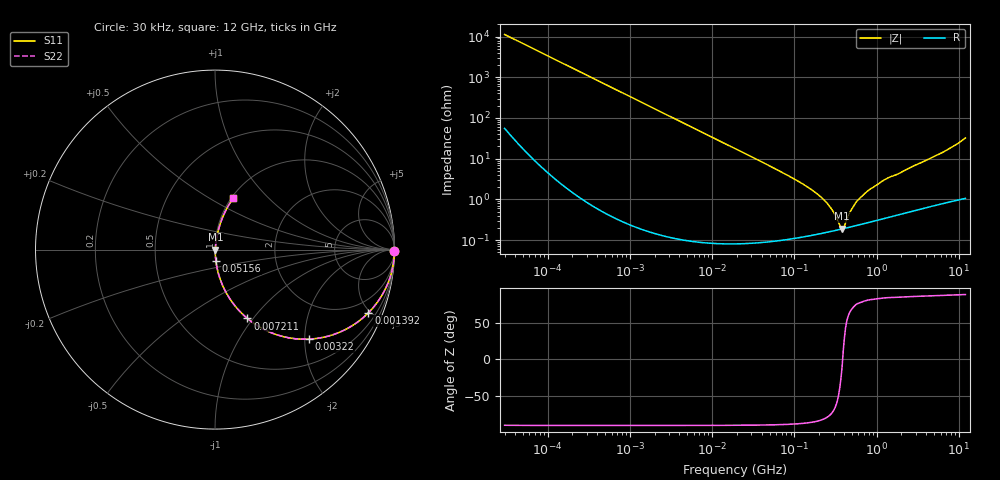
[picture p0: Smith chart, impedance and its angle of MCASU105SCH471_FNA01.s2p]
! MCASU105SCH471_FNA01  S-PARAMETER MODEL  ( General Type )
! Model Generated by TAIYO YUDEN Corporation (http://www.ty-top.com)
! Version 1.0
! TAIYO YUDEN Control No. 130207
! Copyright(c) 2013 TAIYO YUDEN CO.,LTD. All Rights Reserved.
! Product Description (link to TY-COMPAS)
! https://ds.yuden.co.jp/TYCOMPAS/or/detail?pn=MCASU105SCH471JFNA01&u=M
! Products Name : Multilayer Ceramic Capacitors
! Characteristics :
!  Capacitance : 470 pF , Rated Voltage : 50V , TCC : CH / C0H
!  Case Size : 1.0 x 0.5 / 0.039 x 0.02 [mm/inch] , Thickness : 0.5 / 0.02 [mm/inch]
!  (Conditions: Temperature = 25 degC , DC Bias Current/Voltage = 0A / 0V)
! External Node Assignments :
!  1  o---| |---o  2
! GND o---------o GND
! Frequency Range : 30000Hz  -  12GHz  [ 401 STEP ]
# MHz S RI R 50
! Freq[MHz].  S11 Real  S11 Imag  S21 Real  S21 Imag  S12 Real  S12 Imag  S22 Real  S22 Imag
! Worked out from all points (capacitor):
!   401 points, 30 kHz to 12 GHz, reference 50 ohm
!   read as one part in series: C = 471 pF near 32 kHz
!   lowest |Z| = 191 mohm at 380.7 MHz (marker M1)
!   series resonance near 386.2 MHz, so ESL is about 360 pH
!   S11 on the Smith chart (normalised r, x): 30 kHz: open; 1.392 MHz: 1.00, -4.86; 3.22 MHz: 1.00, -2.10; 7.211 MHz: 1.00, -0.94; 51.56 MHz: 1.00, -0.13; 12 GHz: 1.02, +0.65
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0.03  0.9999 -0.00887  0.000122 0.00887  0.000122 0.00887  0.9999 -0.00887
0.260295  0.994 -0.0765  0.00595 0.0765  0.00595 0.0765  0.994 -0.0765
0.730518  0.9553 -0.2064  0.0447 0.2064  0.0447 0.2064  0.9553 -0.2064
1.392304  0.8548 -0.3519  0.1452 0.3519  0.1452 0.3519  0.8548 -0.3519
2.258455  0.6913 -0.4615  0.3087 0.4615  0.3087 0.4615  0.6913 -0.4615
3.22009  0.5243 -0.4989  0.4757 0.4989  0.4757 0.4989  0.5243 -0.4989
7.211021  0.1806 -0.3837  0.8194 0.3837  0.8194 0.3837  0.1806 -0.3837
10.96639  0.0873 -0.2809  0.9127 0.2809  0.9127 0.2809  0.0873 -0.2809
18.97367  0.0314 -0.1721  0.9686 0.1721  0.9686 0.1721  0.0314 -0.1721
51.55976  0.00504 -0.064  0.995 0.064  0.995 0.064  0.00504 -0.064
164.6252  0.00159 -0.0168  0.9984 0.0168  0.9984 0.0168  0.00159 -0.0168
258.5642  0.00163 -0.00723  0.9984 0.00723  0.9984 0.00723  0.00163 -0.00723
303.8045  0.00171 -0.00428  0.9983 0.00428  0.9983 0.00428  0.00171 -0.00428
356.9603  0.00182 -0.00143  0.9982 0.00143  0.9982 0.00143  0.00182 -0.00143
380.7415  0.00188 -0.000322  0.9981 0.000322  0.9981 0.000322  0.00188 -0.000322
406.107  0.00193 0.0011  0.9981 -0.0011  0.9981 -0.0011  0.00193 0.0011
492.8008  0.00215 0.00512  0.9979 -0.00512  0.9979 -0.00512  0.00215 0.00512
598.0015  0.00242 0.00943  0.9976 -0.00943  0.9976 -0.00943  0.00242 0.00943
799.3715  0.00297 0.0165  0.997 -0.0165  0.997 -0.0165  0.00297 0.0165
1428.372  0.00483 0.0344  0.9952 -0.0344  0.9952 -0.0344  0.00483 0.0344
5534.236  0.0223 0.1211  0.9777 -0.1211  0.9777 -0.1211  0.0223 0.1211
12000  0.102 0.2867  0.898 -0.2867  0.898 -0.2867  0.102 0.2867
